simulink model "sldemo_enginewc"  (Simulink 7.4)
settings: Solver=ode23s  SolverMode=SingleTasking  StartTime=0.0  StopTime=10  RelTol=1e-3  AbsTol=1e-6
PreLoadFcn:
  | Kp =0.0614; Ki = 0.0723;
model workspace: external: M-Code (data not in the file)
undefined symbols (not defined in the file or in its folder): DiscIntNeverNeededParam

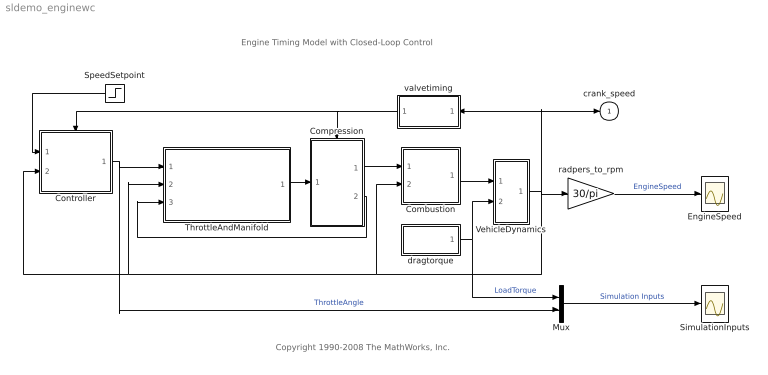
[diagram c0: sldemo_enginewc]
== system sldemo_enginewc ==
  note: Engine Timing Model with Closed-Loop Control
  note: Copyright 1990-2008 The MathWorks, Inc.
  Combustion : Subsystem
  Compression : Subsystem  TreatAsAtomicUnit=on
  Controller : Subsystem  TreatAsAtomicUnit=on
  EngineSpeed : Scope
  Mux : Mux  Inputs=2
  SimulationInputs : Scope
  SpeedSetpoint : Step  Description=|  Time=5  Before=2000  After=3000  SampleTime=0
      | begin dimension               
      | OUTPUT _ : [(time minute -1)];
      | end dimension
  ThrottleAndManifold : Subsystem
  VehicleDynamics : Subsystem
  dragtorque : Subsystem
  radpers_to_rpm : Gain  Description=|  Gain=30/pi  ParameterDataType=sfix(16)  ParameterScaling=2^0  OutDataType=sfix(16)  OutScaling=2^0
      | begin dimension              
      | output _ : [(dimensionless)];
      | end dimension
  valvetiming : Subsystem
  crank_speed : Outport  Description=|  OutDataType=sfix(16)  OutScaling=2^0  InitialOutput=0
      | begin dimension              
      | input _ : [(time second -1)];
      | end dimension
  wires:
  SpeedSetpoint/1 -> Controller/1(Desired_rpm)
  dragtorque/1(Load) -> Mux/1, VehicleDynamics/2(Tload)  "LoadTorque"
  Controller/1(ThrottleAng.) -> Mux/2, ThrottleAndManifold/1(ThrottleAngle)  "ThrottleAngle"
  Compression/1(mass_k) -> Combustion/1(AirCharge)
  valvetiming/1(edge180) -> Controller/Trigger, Compression/Trigger
  Combustion/1(Torque) -> VehicleDynamics/1(Teng)
  VehicleDynamics/1(N) -> Controller/2(N), ThrottleAndManifold/2(EngineSpeedN), Combustion/2(N), valvetiming/1(N), crank_speed/1, radpers_to_rpm/1
  radpers_to_rpm/1 -> EngineSpeed/1  "EngineSpeed"
  Mux/1 -> SimulationInputs/1  "Simulation Inputs"
  ThrottleAndManifold/1(mass_kplus1) -> Compression/1(mass_kplus1)
  Compression/2(trigger) -> ThrottleAndManifold/3(trigger)

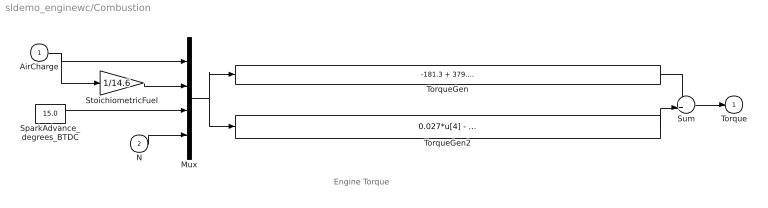
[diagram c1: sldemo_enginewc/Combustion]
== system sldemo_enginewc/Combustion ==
  note: Engine Torque
  AirCharge : Inport  Description=|  OutDataType=sfix(16)  OutScaling=2^0
      | begin dimension            
      | output _ : [(mass gram 1)];
      | end dimension
  N : Inport  Description=|  Port=2  OutDataType=sfix(16)  OutScaling=2^0
      | begin dimension               
      | output _ : [(time second -1)];
      | end dimension
  Mux : Mux
  SparkAdvance_degrees_BTDC : Constant  Value=15.0  OutDataType=sfix(16)  OutScaling=2^0
  StoichiometricFuel : Gain  Gain=1/14.6  ParameterDataType=sfix(16)  ParameterScaling=2^0  OutDataType=sfix(16)  OutScaling=2^0
  Sum : Sum  OutDataType=sfix(16)  OutScaling=2^0
  TorqueGen : Fcn  Description=|  Expr=-181.3 + 379.36*u[1] + 21.91*u[1]/u[2] - (0.85*u[1]*u[1])/(u[2]*u[2]) + 0.26*u[3] - 0.0028*u[3]*u[3]
      | begin dimension                                                      
      | input 1 : [(mass gram 1) | (unknown) | (unknown) | (time second -1)];
      | output 1 : [(length metre 2, mass gram 1, time second -2)];          
      | end dimension
  TorqueGen2 : Fcn  Description=|  Expr=0.027*u[4] - 0.000107*u[4]*u[4] + 0.00048*u[4]*u[3] + 2.55*u[3]*u[1] - 0.05*u[3]*u[3]*u[1]
      | begin dimension                                                      
      | input 1 : [(mass gram 1) | (unknown) | (unknown) | (time second -1)];
      | output 1 : [(length metre 2, mass gram 1, time second -2)];          
      | end dimension
  Torque : Outport  Description=|  OutDataType=sfix(16)  OutScaling=2^0  InitialOutput=0
      | begin dimension                                           
      | input _ : [(length metre 2, mass gram 1, time second -2)];
      | end dimension
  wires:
  StoichiometricFuel/1 -> Mux/2
  SparkAdvance_degrees_BTDC/1 -> Mux/3
  N/1 -> Mux/4
  AirCharge/1 -> StoichiometricFuel/1, Mux/1
  Mux/1 -> TorqueGen/1, TorqueGen2/1
  TorqueGen2/1 -> Sum/2
  TorqueGen/1 -> Sum/1
  Sum/1 -> Torque/1

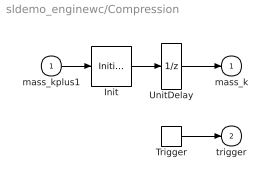
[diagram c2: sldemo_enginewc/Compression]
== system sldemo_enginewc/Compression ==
  mass_kplus1 : Inport  Description=|  OutDataType=sfix(16)  OutScaling=2^0
      | begin dimension            
      | output _ : [(mass gram 1)];
      | end dimension
  Trigger : TriggerPort  TriggerType=either  ShowOutputPort=on
  Init : InitialCondition  Value=0.152
  UnitDelay : UnitDelay  X0=0.152  SampleTime=-1
  mass_k : Outport  Description=|  OutDataType=sfix(16)  OutScaling=2^0  InitialOutput=0.152
      | begin dimension           
      | input _ : [(mass gram 1)];
      | end dimension
  trigger : Outport  Description=|  Port=2  OutDataType=sfix(16)  OutScaling=2^0  InitialOutput=-1
      | begin dimension             
      | input _ : [(dimensionless)];
      | end dimension
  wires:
  Init/1 -> UnitDelay/1
  mass_kplus1/1 -> Init/1
  UnitDelay/1 -> mass_k/1
  Trigger/1 -> trigger/1

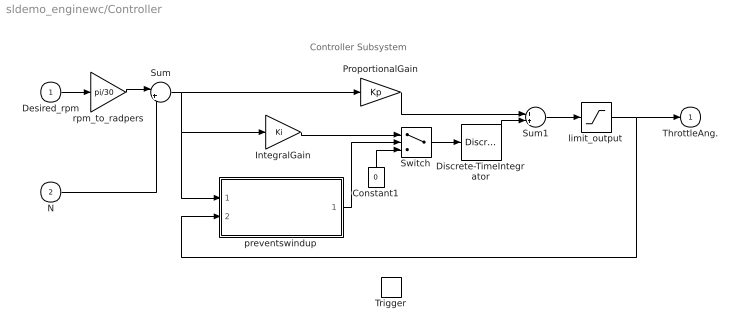
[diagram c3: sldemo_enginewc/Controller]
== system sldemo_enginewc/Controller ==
  note: Controller Subsystem
  Desired_rpm : Inport  Description=|  OutDataType=sfix(16)  OutScaling=2^0
      | begin dimension               
      | output _ : [(time minute -1)];
      | end dimension
  N : Inport  Description=|  Port=2  OutDataType=sfix(16)  OutScaling=2^0
      | begin dimension               
      | output _ : [(time second -1)];
      | end dimension
  Trigger : TriggerPort  TriggerType=either
  Constant1 : Constant  Description=|  Value=0  OutDataType=sfix(16)  OutScaling=2^0
      | begin dimension     
      | output _ : [(zero)];
      | end dimension
  Discrete-TimeIntegrator : DiscreteIntegrator  InitialCondition=8.973  SampleTime=-1  OutDataType=sfix(16)  OutScaling=2^0  ICPrevOutput=DiscIntNeverNeededParam  ICPrevScaledInput=DiscIntNeverNeededParam
  IntegralGain : Gain  Description=|  Gain=Ki  ParameterDataType=sfix(16)  ParameterScaling=2^0  OutDataType=sfix(16)  OutScaling=2^0
      | begin dimension                
      | constant _ : [(dimensionless)];
      | end dimension
  ProportionalGain : Gain  Description=|  Gain=Kp  ParameterDataType=sfix(16)  ParameterScaling=2^0  OutDataType=sfix(16)  OutScaling=2^0
      | begin dimension                
      | constant _ : [(time second 1)];
      | end dimension
  Sum : Sum  Inputs=|+-  OutDataType=sfix(16)  OutScaling=2^0
  Sum1 : Sum  OutDataType=sfix(16)  OutScaling=2^0
  Switch : Switch  Description=|  Threshold=0.5
      | begin dimension              
      | output _ : [(dimensionless)];
      | end dimension
  limit_output : Saturate  UpperLimit=70  LowerLimit=0
  preventswindup : Subsystem
  rpm_to_radpers : Gain  Description=|  Gain=pi/30  ParameterDataType=sfix(16)  ParameterScaling=2^0  OutDataType=sfix(16)  OutScaling=2^0
      | begin dimension                
      | constant _ : [(dimensionless)];
      | end dimension
  ThrottleAng. : Outport  Description=|  OutDataType=sfix(16)  OutScaling=2^0  InitialOutput=8.973
      | begin dimension             
      | input _ : [(dimensionless)];
      | end dimension
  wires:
  rpm_to_radpers/1 -> Sum/1
  Discrete-TimeIntegrator/1 -> Sum1/2
  limit_output/1 -> preventswindup/2(controller_output), ThrottleAng./1
  preventswindup/1(enable_integration) -> Switch/2
  Sum1/1 -> limit_output/1
  Switch/1 -> Discrete-TimeIntegrator/1
  ProportionalGain/1 -> Sum1/1
  Constant1/1 -> Switch/3
  IntegralGain/1 -> Switch/1
  Sum/1 -> preventswindup/1(integrator_input), IntegralGain/1, ProportionalGain/1
  N/1 -> Sum/2
  Desired_rpm/1 -> rpm_to_radpers/1

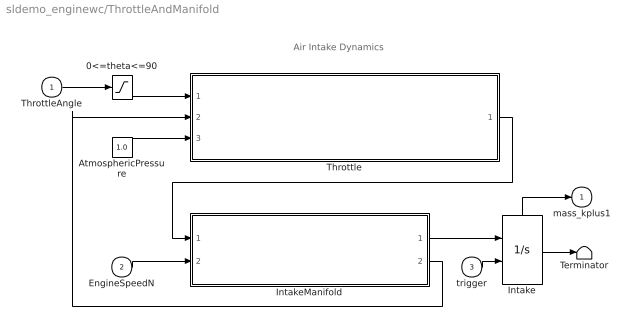
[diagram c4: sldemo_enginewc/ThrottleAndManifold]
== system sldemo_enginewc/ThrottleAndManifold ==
  note: Air Intake Dynamics
  ThrottleAngle : Inport  Description=|  OutDataType=sfix(16)  OutScaling=2^0
      | begin dimension              
      | output _ : [(dimensionless)];
      | end dimension
  EngineSpeedN : Inport  Description=|  Port=2  OutDataType=sfix(16)  OutScaling=2^0
      | begin dimension               
      | output _ : [(time second -1)];
      | end dimension
  trigger : Inport  Description=|  Port=3  OutDataType=sfix(16)  OutScaling=2^0
      | begin dimension              
      | output _ : [(dimensionless)];
      | end dimension
  0<=theta<=90 : Saturate  UpperLimit=90  LowerLimit=0
  AtmosphericPressure : Constant  Description=|  Value=1.0  OutDataType=sfix(16)  OutScaling=2^0
      | begin dimension                                       
      | output _ : [(length bar -1, mass bar 1, time bar -2)];
      | end dimension
  Intake : Integrator  ExternalReset=either  ShowStatePort=on  ZeroCross=off
  IntakeManifold : Subsystem
  Terminator : Terminator
  Throttle : Subsystem
  mass_kplus1 : Outport  Description=|  OutDataType=sfix(16)  OutScaling=2^0  InitialOutput=0
      | begin dimension           
      | input _ : [(mass gram 1)];
      | end dimension
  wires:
  0<=theta<=90/1 -> Throttle/1(ThrottleAngle)
  ThrottleAngle/1 -> 0<=theta<=90/1
  Throttle/1(ThrottleFlow) -> IntakeManifold/1(mdotInput)
  EngineSpeedN/1 -> IntakeManifold/2(N)
  IntakeManifold/2(ManifoldPressure_Pm) -> Throttle/2(ManifoldPressure)
  IntakeManifold/1(mdot_to_Cylinder) -> Intake/1
  AtmosphericPressure/1 -> Throttle/3(AtmosphericPressure)
  trigger/1 -> Intake/2
  Intake/1 -> Terminator/1
  Intake/State -> mass_kplus1/1

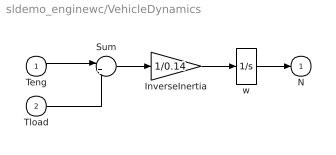
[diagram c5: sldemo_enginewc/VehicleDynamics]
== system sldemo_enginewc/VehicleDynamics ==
  Teng : Inport  Description=|  OutDataType=sfix(16)  OutScaling=2^0
      | begin dimension                                            
      | output _ : [(length metre 2, mass gram 1, time second -2)];
      | end dimension
  Tload : Inport  Description=|  Port=2  OutDataType=sfix(16)  OutScaling=2^0
      | begin dimension                                            
      | output _ : [(length metre 2, mass gram 1, time second -2)];
      | end dimension
  InverseInertia : Gain  Description=|  Gain=1/0.14  ParameterDataType=sfix(16)  ParameterScaling=2^0  OutDataType=sfix(16)  OutScaling=2^0
      | begin dimension                                
      | constant _ : [(length metre -2, mass gram -1)];
      | end dimension
  Sum : Sum  Inputs=|+-  OutDataType=sfix(16)  OutScaling=2^0
  w : Integrator  InitialCondition=209.48
  N : Outport  Description=|  OutDataType=sfix(16)  OutScaling=2^0  InitialOutput=0
      | begin dimension              
      | input _ : [(time second -1)];
      | end dimension
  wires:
  InverseInertia/1 -> w/1
  w/1 -> N/1
  Sum/1 -> InverseInertia/1
  Teng/1 -> Sum/1
  Tload/1 -> Sum/2

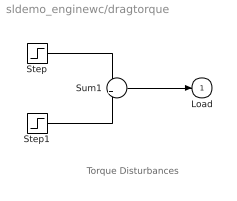
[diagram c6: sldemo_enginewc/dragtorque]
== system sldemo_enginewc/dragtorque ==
  note: Torque Disturbances
  Step : Step  Description=|  Time=2  Before=25  After=20  SampleTime=0
      | begin dimension                                            
      | output _ : [(length metre 2, mass gram 1, time second -2)];
      | end dimension
  Step1 : Step  Description=|  Time=8  After=5  SampleTime=0
      | begin dimension                                            
      | output _ : [(length metre 2, mass gram 1, time second -2)];
      | end dimension
  Sum1 : Sum  OutDataType=sfix(16)  OutScaling=2^0
  Load : Outport  Description=|  OutDataType=sfix(16)  OutScaling=2^0  InitialOutput=0
      | begin dimension                                           
      | input _ : [(length metre 2, mass gram 1, time second -2)];
      | end dimension
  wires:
  Sum1/1 -> Load/1
  Step/1 -> Sum1/1
  Step1/1 -> Sum1/2

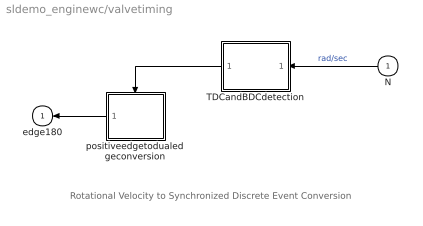
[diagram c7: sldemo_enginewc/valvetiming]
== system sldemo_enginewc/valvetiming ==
  note: Rotational Velocity to Synchronized Discrete Event Conversion
  N : Inport  Description=|  OutDataType=sfix(16)  OutScaling=2^0
      | begin dimension               
      | output _ : [(time second -1)];
      | end dimension
  TDCandBDCdetection : Subsystem
  positiveedgetodualedgeconversion : Subsystem  TreatAsAtomicUnit=on
  edge180 : Outport  Description=|  OutDataType=sfix(16)  OutScaling=2^0  InitialOutput=-1
      | begin dimension             
      | input _ : [(dimensionless)];
      | end dimension
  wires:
  TDCandBDCdetection/1(trigger) -> positiveedgetodualedgeconversion/Trigger
  positiveedgetodualedgeconversion/1(trigger) -> edge180/1
  N/1 -> TDCandBDCdetection/1(N)  "rad/sec"

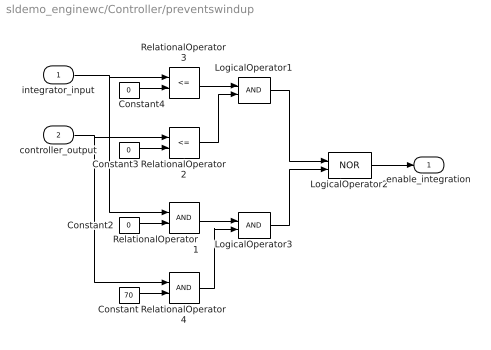
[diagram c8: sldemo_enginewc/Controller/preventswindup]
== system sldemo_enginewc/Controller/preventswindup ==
  integrator_input : Inport  Description=|  OutDataType=sfix(16)  OutScaling=2^0
      | begin dimension               
      | output _ : [(time second -1)];
      | end dimension
  controller_output : Inport  Description=|  Port=2  OutDataType=sfix(16)  OutScaling=2^0
      | begin dimension              
      | output _ : [(dimensionless)];
      | end dimension
  Constant : Constant  Description=|  Value=70  OutDataType=sfix(16)  OutScaling=2^0
      | begin dimension              
      | output _ : [(dimensionless)];
      | end dimension
  Constant2 : Constant  Description=|  Value=0  OutDataType=sfix(16)  OutScaling=2^0
      | begin dimension     
      | output _ : [(zero)];
      | end dimension
  Constant3 : Constant  Description=|  Value=0  OutDataType=sfix(16)  OutScaling=2^0
      | begin dimension     
      | output _ : [(zero)];
      | end dimension
  Constant4 : Constant  Description=|  Value=0  OutDataType=sfix(16)  OutScaling=2^0
      | begin dimension     
      | output _ : [(zero)];
      | end dimension
  LogicalOperator1 : Logic  IconShape=distinctive
  LogicalOperator2 : Logic  Operator=NOR  IconShape=distinctive
  LogicalOperator3 : Logic  IconShape=distinctive
  RelationalOperator1 : RelationalOperator
  RelationalOperator2 : RelationalOperator  Operator=<=
  RelationalOperator3 : RelationalOperator  Operator=<=
  RelationalOperator4 : RelationalOperator
  enable_integration : Outport  Description=|  OutDataType=sfix(16)  OutScaling=2^0  InitialOutput=0
      | begin dimension             
      | input _ : [(dimensionless)];
      | end dimension
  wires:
  LogicalOperator2/1 -> enable_integration/1
  LogicalOperator3/1 -> LogicalOperator2/2
  LogicalOperator1/1 -> LogicalOperator2/1
  RelationalOperator4/1 -> LogicalOperator3/2
  RelationalOperator1/1 -> LogicalOperator3/1
  Constant/1 -> RelationalOperator4/2
  Constant2/1 -> RelationalOperator1/2
  controller_output/1 -> RelationalOperator4/1, RelationalOperator2/1
  integrator_input/1 -> RelationalOperator3/1, RelationalOperator1/1
  RelationalOperator2/1 -> LogicalOperator1/2
  RelationalOperator3/1 -> LogicalOperator1/1
  Constant4/1 -> RelationalOperator3/2
  Constant3/1 -> RelationalOperator2/2

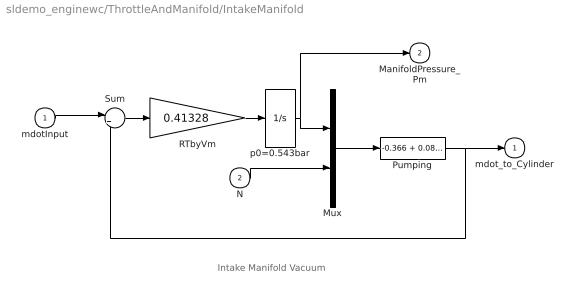
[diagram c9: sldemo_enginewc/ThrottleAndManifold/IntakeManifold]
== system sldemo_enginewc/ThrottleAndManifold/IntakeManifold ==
  note: Intake Manifold Vacuum
  mdotInput : Inport  Description=|  OutDataType=sfix(16)  OutScaling=2^0
      | begin dimension                            
      | output _ : [(mass gram 1, time second -1)];
      | end dimension
  N : Inport  Description=|  Port=2  OutDataType=sfix(16)  OutScaling=2^0
      | begin dimension               
      | output _ : [(time second -1)];
      | end dimension
  Mux : Mux  Inputs=2
  Pumping : Fcn  Description=|  Expr=-0.366 + 0.08979*u[1]*u[2] - 0.0337*u[2]*u[1]*u[1] + 0.0001*u[1]*u[2]*u[2]
      | begin dimension                                                         
      | input 1 : [(length bar -1, mass bar 1, time bar -2) | (time second -1)];
      | output 1 : [(mass gram 1, time second -1)];                             
      | end dimension
  RTbyVm : Gain  Description=|  Gain=0.41328  ParameterDataType=sfix(16)  ParameterScaling=2^0  OutDataType=sfix(16)  OutScaling=2^0
      | begin dimension                                  
      | constant _ : [(length metre -1, time second -2)];
      | end dimension
  Sum : Sum  Inputs=|+-  OutDataType=sfix(16)  OutScaling=2^0
  p0=0.543bar : Integrator  InitialCondition=.543
  mdot_to_Cylinder : Outport  Description=|  OutDataType=sfix(16)  OutScaling=2^0  InitialOutput=0
      | begin dimension                           
      | input _ : [(mass gram 1, time second -1)];
      | end dimension
  ManifoldPressure_Pm : Outport  Description=|  Port=2  OutDataType=sfix(16)  OutScaling=2^0  InitialOutput=0
      | begin dimension                                      
      | input _ : [(length bar -1, mass bar 1, time bar -2)];
      | end dimension
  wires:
  mdotInput/1 -> Sum/1
  RTbyVm/1 -> p0=0.543bar/1
  N/1 -> Mux/2
  Mux/1 -> Pumping/1
  p0=0.543bar/1 -> Mux/1, ManifoldPressure_Pm/1
  Sum/1 -> RTbyVm/1
  Pumping/1 -> Sum/2, mdot_to_Cylinder/1

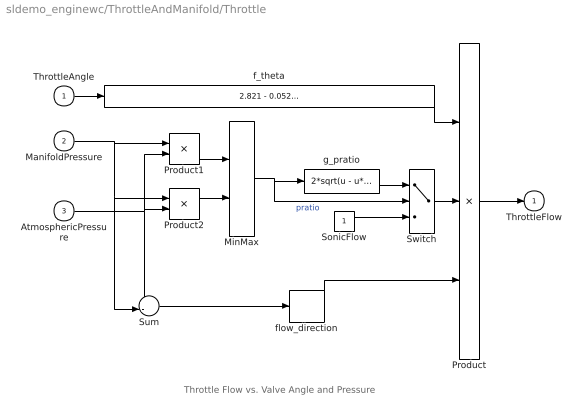
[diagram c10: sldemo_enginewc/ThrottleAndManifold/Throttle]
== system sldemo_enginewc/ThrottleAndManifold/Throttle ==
  note: Throttle Flow vs. Valve Angle and Pressure
  ThrottleAngle : Inport  Description=|  OutDataType=sfix(16)  OutScaling=2^0
      | begin dimension              
      | output _ : [(dimensionless)];
      | end dimension
  ManifoldPressure : Inport  Description=|  Port=2  OutDataType=sfix(16)  OutScaling=2^0
      | begin dimension                                       
      | output _ : [(length bar -1, mass bar 1, time bar -2)];
      | end dimension
  AtmosphericPressure : Inport  Description=|  Port=3  OutDataType=sfix(16)  OutScaling=2^0
      | begin dimension                                       
      | output _ : [(length bar -1, mass bar 1, time bar -2)];
      | end dimension
  MinMax : MinMax  Inputs=2  OutDataType=sfix(16)  OutScaling=2^0
  Product : Product  Inputs=3  OutDataType=sfix(16)  OutScaling=2^0
  Product1 : Product  Inputs=*/  OutDataType=sfix(16)  OutScaling=2^0
  Product2 : Product  Inputs=/*  OutDataType=sfix(16)  OutScaling=2^0
  SonicFlow : Constant  Description=|  OutDataType=sfix(16)  OutScaling=2^0
      | begin dimension              
      | output _ : [(dimensionless)];
      | end dimension
  Sum : Sum  Inputs=+-|  OutDataType=sfix(16)  OutScaling=2^0
  Switch : Switch  Description=|  Threshold=0.5
      | begin dimension                 
      | threshold _ : [(dimensionless)];
      | end dimension
  f_theta : Fcn  Description=|  Expr=2.821 - 0.05231*u + 0.10299*u*u - 0.00063*u*u*u
      | begin dimension             
      | input 1 : [(dimensionless)];
      | output 1 : [(unknown)];     
      | end dimension
  flow_direction : Signum
  g_pratio : Fcn  Description=|  Expr=2*sqrt(u - u*u)
      | begin dimension              
      | input 1 : [(dimensionless)]; 
      | output 1 : [(dimensionless)];
      | end dimension
  ThrottleFlow : Outport  Description=|  OutDataType=sfix(16)  OutScaling=2^0  InitialOutput=0
      | begin dimension                           
      | input _ : [(mass gram 1, time second -1)];
      | end dimension
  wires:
  ManifoldPressure/1 -> Sum/2, Product2/1, Product1/1
  Product2/1 -> MinMax/2
  Product1/1 -> MinMax/1
  AtmosphericPressure/1 -> Sum/1, Product2/2, Product1/2
  g_pratio/1 -> Switch/1
  SonicFlow/1 -> Switch/3
  Switch/1 -> Product/2
  flow_direction/1 -> Product/3
  Sum/1 -> flow_direction/1
  MinMax/1 -> Switch/2, g_pratio/1  "pratio"
  ThrottleAngle/1 -> f_theta/1
  Product/1 -> ThrottleFlow/1
  f_theta/1 -> Product/1

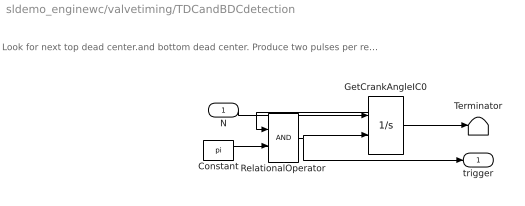
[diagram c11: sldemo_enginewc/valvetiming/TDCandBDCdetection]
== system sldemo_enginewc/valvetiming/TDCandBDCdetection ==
  note: Look for next top dead center.and bottom dead center. Produce two pulses per revolution.
  N : Inport  Description=|  OutDataType=sfix(16)  OutScaling=2^0
      | begin dimension               
      | output _ : [(time second -1)];
      | end dimension
  Constant : Constant  Description=|  Value=pi  OutDataType=sfix(16)  OutScaling=2^0
      | begin dimension              
      | output _ : [(dimensionless)];
      | end dimension
  GetCrankAngleIC0 : Integrator  ExternalReset=rising  ShowStatePort=on
  RelationalOperator : RelationalOperator
  Terminator : Terminator
  trigger : Outport  Description=|  OutDataType=sfix(16)  OutScaling=2^0  InitialOutput=0
      | begin dimension             
      | input _ : [(dimensionless)];
      | end dimension
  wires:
  N/1 -> GetCrankAngleIC0/1
  RelationalOperator/1 -> trigger/1, GetCrankAngleIC0/2
  Constant/1 -> RelationalOperator/2
  GetCrankAngleIC0/State -> RelationalOperator/1
  GetCrankAngleIC0/1 -> Terminator/1

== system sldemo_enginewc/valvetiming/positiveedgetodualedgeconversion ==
  Trigger : TriggerPort
  Gain : Gain  Description=|  Gain=-1  ParameterDataType=sfix(16)  ParameterScaling=2^0  OutDataType=sfix(16)  OutScaling=2^0
      | begin dimension                
      | constant _ : [(dimensionless)];
      | end dimension
  UnitDelay : UnitDelay  X0=1  SampleTime=-1
  trigger : Outport  Description=|  OutDataType=sfix(16)  OutScaling=2^0  InitialOutput=-1
      | begin dimension             
      | input _ : [(dimensionless)];
      | end dimension
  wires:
  Gain/1 -> UnitDelay/1
  UnitDelay/1 -> trigger/1, Gain/1
